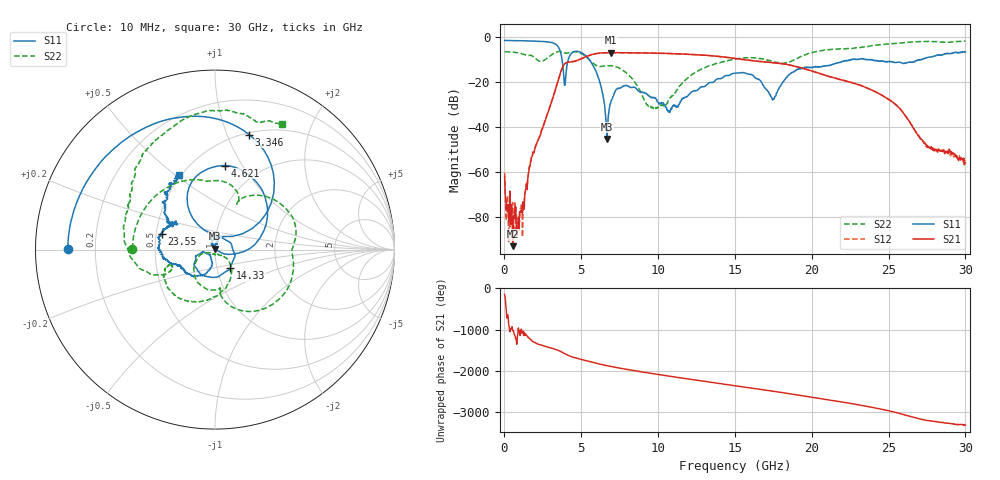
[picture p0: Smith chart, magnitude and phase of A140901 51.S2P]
!  2-Port S-parameters saved by WinCal
! VAR MeasName=S-Parameters (CALIBRATED_DATA) read from VNA (N5244A)
! VAR MeasDate=11/3/2014 9:35:54 AM
! VAR NAME=A140901 51
! VAR FILENAME=A140901 51.S2P
! VAR DATE=11/3/2014 9:35:54 AM
! VAR PHYS_PORTS=1,2
# Hz S RI R 50
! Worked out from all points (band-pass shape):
!   801 points, 10 MHz to 30 GHz, reference 50 ohm
!   highest |S21| = -7.10 dB at 6.908 GHz (marker M1); lowest = -92.9 dB at 534.8 MHz (marker M2)
!   |S21| within 3 dB of the highest: 4.902 GHz to 15.49 GHz (10.59 GHz wide, 104 % of centre)
!   lowest |S11| = -45.4 dB at 6.683 GHz (marker M3), VSWR 1.01, Z = 50.1 + j0.518 ohm
!   |S11| at or under -10 dB: 3.745 GHz to 4.163 GHz (418 MHz wide, 10.6 % of centre); 5.493 GHz to 22.69 GHz (17.19 GHz wide, 122 % of centre); 23.42 GHz to 27.23 GHz (3.814 GHz wide, 15.1 % of centre)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
!   |S22| runs from -32.0 to -2.0 dB; largest |S21 - S12| = 0.0032
!   S11 on the Smith chart (normalised r, x): 10 MHz: 0.10, +0.00; 3.346 GHz: 0.52, +1.20; 4.621 GHz: 0.70, +0.84; 14.33 GHz: 1.16, -0.24; 23.55 GHz: 0.54, +0.10; 30 GHz: 0.49, +0.52
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1e7  -0.8194 0.00365  -0.000686 -0.000424  -0.000536 -0.000811  -0.4601 0.00466
5.34825e8  -0.7984 0.1737  1.08e-05 2e-05  4.94e-05 0.000204  -0.3799 0.2447
1.134625e9  -0.726 0.3583  0.000141 3.33e-06  0.000184 7.08e-05  -0.1548 0.3857
1.771912e9  -0.5915 0.5363  -0.00215 0.000154  -0.00224 0.000152  0.0657 0.3729
3.346388e9  0.19 0.6409  0.0582 -0.0437  0.0582 -0.0437  0.3646 0.2552
3.946188e9  -0.0129 0.085  -0.2049 -0.1486  -0.2049 -0.1485  0.4301 0.00424
4.620962e9  0.0544 0.4679  -0.1465 0.2467  -0.1467 0.2463  0.3978 -0.2288
5.033325e9  0.2452 0.3579  0.0596 0.3217  0.0593 0.3213  0.2424 -0.3391
6.045488e9  0.1416 -0.016  0.4074 -0.1153  0.4076 -0.1149  0.0295 -0.2193
6.682775e9  0.00141 0.00516  0.1616 -0.4083  0.1616 -0.4075  -0.00159 -0.2248
6.9077e9  -0.0192 0.0278  0.0322 -0.4405  0.0325 -0.4393  -0.033 -0.2243
8.332225e9  0.0144 0.0731  -0.4372 0.0116  -0.4367 0.0107  -0.101 -0.0564
1.001916e10  0.00909 0.0331  0.0871 0.4197  0.0867 0.419  -0.00228 -0.0273
1.163112e10  -0.0182 0.0399  0.4012 -0.0812  0.4016 -0.0809  0.0748 -0.0598
1.433022e10  0.0856 -0.1014  -0.3255 -0.1288  -0.3258 -0.1294  -0.0396 -0.2785
1.5005e10  -6.71e-05 -0.1538  -0.3174 0.0803  -0.3169 0.0805  -0.1239 -0.2913
1.747918e10  -0.0296 -0.0283  0.2143 0.1529  0.214 0.154  -0.2625 -0.0915
2.002832e10  -0.1786 -0.1058  -0.0681 -0.1571  -0.0672 -0.1581  -0.434 -0.0885
2.355215e10  -0.2946 0.0882  0.0632 0.0372  0.0634 0.0372  -0.4574 0.3823
2.501416e10  -0.2315 0.1489  0.00774 -0.0395  0.00781 -0.0396  -0.3416 0.6006
2.76008e10  -0.2819 0.2027  0.00248 0.00258  0.00267 0.00238  0.067 0.7784
3e10  -0.1985 0.4155  0.000609 -0.00148  0.000667 -0.0017  0.3756 0.7002
